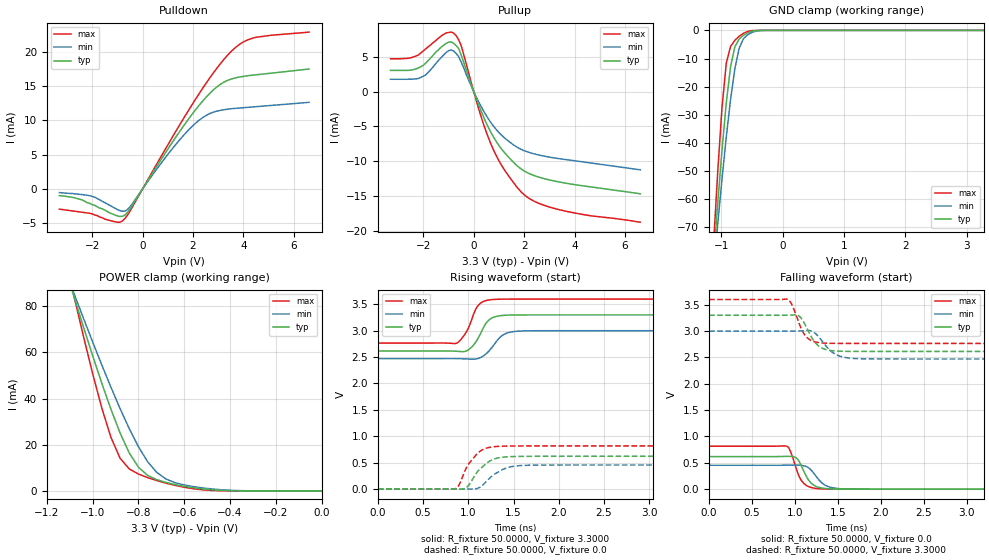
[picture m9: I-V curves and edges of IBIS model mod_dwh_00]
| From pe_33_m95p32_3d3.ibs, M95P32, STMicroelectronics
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|   Model mod_dwh_00
[Model]   mod_dwh_00
Model_type I/O
Polarity   Non-Inverting
Vinl   =   1.000V
Vinh   =   2.300V
Vmeas  =   1.650V
Cref   =   30pF
C_comp   1.607pF   1.535pF   1.683pF
[Model Spec]
Vinl   1.000V  0.900V  1.080V  | <- for Vcc = 3.3V, 3.0V, 3.6V
Vinh   2.300V  2.100V  2.520V  | <- for Vcc = 3.3V, 3.0V, 3.6V
Vmeas  1.650V  1.500V  1.800V  | <- for Vcc = 3.3V, 3.0V, 3.6V
[Temperature Range]   25.0000   0.1050k   -40.0000
[Voltage Range]   3.3000V   3.0000V   3.6000V
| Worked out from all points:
|   slope of the pulldown table from 0 to 0.495 V, typ, clamps not added: 170 ohm
|   slope of the pullup table from 0 to 0.495 V, typ, clamps not added: 110 ohm
|   GND clamp passes 1 mA (typ) near -0.58 V on its own axis
|   POWER clamp passes 1 mA (typ) near -0.53 V on its own axis
|   rising waveform, R_fixture 50.0000, V_fixture 3.3000: 20-80 % time 138ps typ, 158ps min, 130ps max; typ from 2.61 V to 3.3 V
|   rising waveform, R_fixture 50.0000, V_fixture 0.0: 20-80 % time 182ps typ, 203ps min, 169ps max; typ from 0 V to 0.619 V
|   falling waveform, R_fixture 50.0000, V_fixture 0.0: 20-80 % time 125ps typ, 149ps min, 113ps max; typ from 0.619 V to 0 V
|   falling waveform, R_fixture 50.0000, V_fixture 3.3000: 20-80 % time 149ps typ, 181ps min, 130ps max; typ from 3.3 V to 2.61 V
[Pulldown]
|Voltage   I(typ)   I(min)   I(max)
-3.3V     -990uA     -543uA     -2.95mA
-1.9V     -2.4mA     -1.2mA     -3.8mA
-1.1V     -3.8mA     -2.8mA     -4.78mA
-800mV    -4.004mA   -3.256mA   -4.673mA
-500mV    -2.938mA   -2.618mA   -3.241mA
1V        5.787mA    5.02mA     6.403mA
2V        11.05mA    9.22mA     12.48mA
2.8V      14.39mA    11.16mA    16.86mA
3.5V      15.98mA    11.66mA    19.96mA
4V        16.38mA    11.82mA    21.4mA
4.5V      16.61mA    11.97mA    22.07mA
6.6V      17.45mA    12.62mA    22.83mA
[Pullup]
|Voltage   I(typ)   I(min)   I(max)
-3.3V     3.03mA     1.76mA     4.701mA
-2.1V     3.543mA    2.023mA    5.511mA
-1.1V     6.877mA    5.565mA    8.378mA
-800mV    6.924mA    5.82mA     8.384mA
-500mV    5.255mA    4.257mA    6.625mA
200mV     -1.954mA   -1.496mA   -2.519mA
700mV     -5.972mA   -4.551mA   -7.671mA
1.2V      -8.668mA   -6.571mA   -11.13mA
1.9V      -11.15mA   -8.323mA   -14.46mA
2.4V      -12.05mA   -8.941mA   -15.73mA
3.3V      -12.9mA    -9.574mA   -16.85mA
6.6V      -14.66mA   -11.22mA   -18.73mA
[GND_clamp]
|Voltage   I(typ)   I(min)   I(max)
-3.3V     -807.6mA   -672mA     -1.053A
-1.13V    -81.94mA   -85.75mA   -76.94mA
-1.06V    -61.58mA   -68.96mA   -50.51mA
-990mV    -42.58mA   -52.9mA    -27.53mA
-920mV    -25.81mA   -37.91mA   -11.64mA
-850mV    -12.88mA   -24.52mA   -5.709mA
-780mV    -5.82mA    -13.61mA   -3.523mA
-710mV    -3.106mA   -6.377mA   -2.091mA
-640mV    -1.742mA   -2.986mA   -1.046mA
-500mV    -309.6uA   -721.8uA   -69.16uA
-290mV    -791nA     -10.61uA   -17.06nA
3.28V     561.4pA    18.21uA    173.1pA
[POWER_clamp]
|Voltage   I(typ)   I(min)   I(max)
-3.28V    853.2mA    705.5mA    1.123A
-1.08V    83.64mA    85.1mA     83.66mA
-1V       58.53mA    64.51mA    50.75mA
-960mV    46.59mA    54.53mA    35.87mA
-920mV    35.3mA     44.85mA    23.13mA
-880mV    25.04mA    35.59mA    14.12mA
-840mV    16.42mA    26.93mA    9.512mA
-800mV    10.26mA    19.14mA    7.302mA
-720mV    4.876mA    8.001mA    4.493mA
-640mV    2.758mA    3.578mA    2.397mA
-400mV    94.29uA    284.7uA    12.64uA
0V        840.7pA    17.31nA    345.8pA
[Ramp]
| variable   typ   min   max
dV/dt_r   0.3712/0.2044n   0.2812/0.2772n   0.4891/0.2510n
dV/dt_f   0.4118/0.2377n   0.3276/0.2560n   0.5005/0.2490n
R_load = 50.0000
[Rising Waveform]
R_fixture= 50.0000
V_fixture= 3.3000
V_fixture_min= 3.0000
V_fixture_max= 3.6000
|time   V(typ)   V(min)   V(max)
0s        2.614V     2.471V     2.766V
872ps     2.61V      2.47V      2.765V
1ns       2.637V     2.463V     3.049V
1.08ns    2.779V     2.462V     3.402V
1.112ns   2.869V     2.475V     3.485V
1.208ns   3.168V     2.58V      3.577V
1.288ns   3.261V     2.743V     3.593V
1.416ns   3.294V     2.948V     3.599V
1.64ns    3.3V       2.997V     3.6V
8ns       3.3V       3V         3.6V
[Rising Waveform]
R_fixture= 50.0000
V_fixture= 0.0
V_fixture_min= 0.0
V_fixture_max= 0.0
|time   V(typ)   V(min)   V(max)
0s        11.55nV    1.186uV    2.101nV
856ps     -948.3uV   276.3uV    437.8uV
896ps     -2.761mV   120.3uV    70.77mV
976ps     21.54mV    -1.309mV   393.5mV
1.104ns   332.8mV    12.45mV    677.9mV
1.232ns   523.6mV    199.4mV    786.9mV
1.328ns   587.2mV    319mV      806.5mV
1.488ns   613.7mV    425.6mV    814mV
1.744ns   618.4mV    451.6mV    815.1mV
8ns       618.7mV    453.5mV    815.2mV
[Falling Waveform]
R_fixture= 50.0000
V_fixture= 0.0
V_fixture_min= 0.0
V_fixture_max= 0.0
|time   V(typ)   V(min)   V(max)
0s        618.7mV    453.5mV    815.2mV
904ps     622.9mV    454.8mV    816.7mV
952ps     622.1mV    456.2mV    702.7mV
1.008ns   602.4mV    457.5mV    426.2mV
1.08ns    424.9mV    450.6mV    152.9mV
1.176ns   137.2mV    383.8mV    38.01mV
1.288ns   30.21mV    161.2mV    7.711mV
1.416ns   5.504mV    34.67mV    1.278mV
1.656ns   249.5uV    1.958mV    50.44uV
8ns       664.6nV    1.827uV    767.8nV
[Falling Waveform]
R_fixture= 50.0000
V_fixture= 3.3000
V_fixture_min= 3.0000
V_fixture_max= 3.6000
|time   V(typ)   V(min)   V(max)
0s        3.3V       3V         3.6V
904ps     3.3V       3V         3.608V
960ps     3.304V     3V         3.517V
1.04ns    3.296V     3.002V     3.186V
1.12ns    3.118V     3.008V     2.916V
1.232ns   2.79V      2.964V     2.796V
1.328ns   2.668V     2.787V     2.773V
1.488ns   2.621V     2.548V     2.767V
1.76ns    2.614V     2.475V     2.766V
8ns       2.614V     2.471V     2.766V
